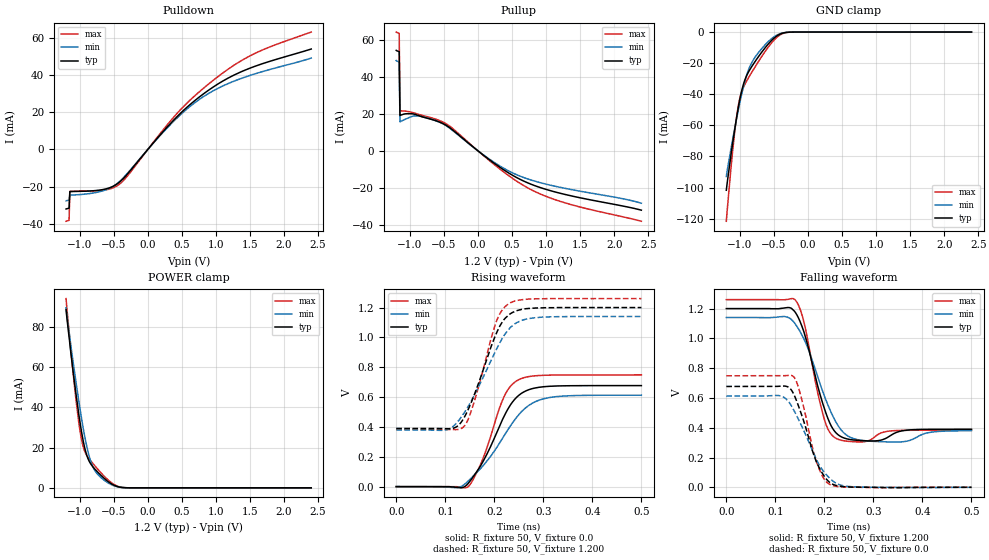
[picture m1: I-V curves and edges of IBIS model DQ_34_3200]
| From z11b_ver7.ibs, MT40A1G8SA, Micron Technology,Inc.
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| MODEL DQ_34_3200 (34 Ohm Data I/O with no ODT, 1600-3200Mbps)
[Model]   DQ_34_3200
Model_type   I/O
Vinl = 905.000mV
Vinh = 1015.000mV
Vmeas = 960.000mV
Vref = 1200.000mV
Cref = 0.0pF
Rref = 50.000Ohm
|   typ   min   max
|C_comp   0.810pF   0.760pF   0.860pF
C_comp_pullup   0.4050pF   0.3800pF   0.4300pF
C_comp_pulldown   0.4050pF   0.3800pF   0.4300pF
[Model Spec]
| Timing spec test load voltage corners
Vref   1.2000V   1.1400V   1.2600V
| Dynamic Overshoot Parameters from DDR4 Specification
|D_overshoot_ampl_h   0.40   NA   NA
|D_overshoot_ampl_l   0.40   NA   NA
|D_overshoot_area_h   0.0800n   NA   NA
|D_overshoot_area_l   0.0800n   NA   NA
[Voltage Range]   1.2000V   1.1400V   1.2600V
| Junction Temperature (Ambient temp is 35C typ, 95C min, 0C max)
[Temperature Range]   50.0   110.0   0.0
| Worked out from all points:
|   slope of the pulldown table from 0 to 0.18 V, typ, clamps not added: 23.2 ohm
|   slope of the pullup table from 0 to 0.18 V, typ, clamps not added: 35.1 ohm
|   GND clamp passes 1 mA (typ) near -0.39 V on its own axis
|   POWER clamp passes 1 mA (typ) near -0.48 V on its own axis
|   rising waveform, R_fixture 50, V_fixture 0.0: 20-80 % time 60.5ps typ, 79.7ps min, 47.2ps max; typ from 0 V to 0.677 V
|   falling waveform, R_fixture 50, V_fixture 1.200: 20-80 % time 39ps typ, 50.4ps min, 31.7ps max; typ from 1.2 V to 0.39 V
|   rising waveform, R_fixture 50, V_fixture 1.200: 20-80 % time 54.3ps typ, 69.6ps min, 43.8ps max; typ from 0.39 V to 1.2 V
|   falling waveform, R_fixture 50, V_fixture 0.0: 20-80 % time 41.1ps typ, 52.9ps min, 33.2ps max; typ from 0.677 V to 0 V
[Pulldown]
|   Voltage   I(typ)   I(min)   I(max)
-1.2V     -32.14mA   -27.78mA   -38.76mA
-1.156V   -31.69mA   -27.3mA    -38.27mA
-1.145V   -22.74mA   -24.67mA   -22.62mA
-698.2mV  -21.88mA   -22.71mA   -22.17mA
-545.5mV  -20.46mA   -20.64mA   -21.17mA
-414.5mV  -17.59mA   -17.27mA   -18.66mA
-294.5mV  -13.07mA   -12.67mA   -14.11mA
458.2mV   18.75mA    17.99mA    20.61mA
752.7mV   28.18mA    26.87mA    30.99mA
1.047V    35.72mA    33.3mA     39.78mA
1.571V    44.84mA    40.76mA    51.79mA
2.4V      54.19mA    49.29mA    63.35mA
[GND_clamp]
|   Voltage   I(typ)   I(min)   I(max)
-1.2V     -101.7mA   -92.84mA   -121.7mA
-1.135V   -79.96mA   -75.84mA   -88.92mA
-1.08V    -63.49mA   -62.76mA   -65.41mA
-1.036V   -51.56mA   -52.83mA   -50.65mA
-992.7mV  -41.38mA   -43.57mA   -41.02mA
-927.3mV  -30.76mA   -31.6mA    -33.57mA
-872.7mV  -25.55mA   -24.13mA   -29.29mA
-818.2mV  -21.61mA   -19.01mA   -25.29mA
-621.8mV  -9.66mA    -7.8mA     -11.96mA
-436.4mV  -1.915mA   -1.476mA   -2.607mA
-229.1mV  -17.62uA   -20.1uA    -21.35uA
2.4V      0A         0A         0A
[Pullup]
|   Voltage   I(typ)   I(min)   I(max)
-1.2V     54.34mA    48.83mA    64.24mA
-1.156V   53.69mA    48.13mA    63.57mA
-1.145V   19.17mA    15.69mA    21.61mA
-916.4mV  19.61mA    18.89mA    20.24mA
-567.3mV  15.61mA    15.52mA    16.42mA
-370.9mV  11.29mA    10.99mA    12.08mA
0V        840nA      835.9nA    929.5nA
327.3mV   -9.01mA    -8.316mA   -9.985mA
589.1mV   -14.86mA   -13.25mA   -16.89mA
861.8mV   -19.2mA    -16.69mA   -22.46mA
1.418V    -24.76mA   -21.28mA   -29.6mA
2.4V      -32.09mA   -28.34mA   -38.11mA
[POWER_clamp]
|   Voltage   I(typ)   I(min)   I(max)
-1.2V     88.79mA    89.61mA    94.2mA
-1.135V   68.71mA    72.12mA    70.03mA
-1.058V   47.63mA    53.55mA    44.95mA
-1.004V   34.46mA    41.11mA    30.27mA
-960mV    25.41mA    31.92mA    21.99mA
-894.5mV  16.02mA    20.41mA    16.03mA
-850.9mV  12.63mA    14.54mA    13.97mA
-807.3mV  10.5mA     10.53mA    12.15mA
-709.1mV  6.91mA     5.769mA    8.279mA
-545.5mV  2.224mA    1.735mA    2.842mA
-305.5mV  24.75uA    26.66uA    31.49uA
2.4V      0A         0A         0A
[Ramp]
|   typ   min   max
dV/dt_r   406.22m/60.49p   367.64m/79.70p   449.27m/47.23p
dV/dt_f   486.12m/38.95p   456.09m/50.39p   526.01m/31.70p
R_load = 50
[Rising Waveform]
R_fixture = 50
V_fixture = 0.0
|   Time   V(typ)   V(min)   V(max)
0s        2.16uV     7.745uV    1.281uV
124ps     -5.863mV   -6.685mV   -787.9uV
147ps     22.02mV    37.71mV    729.1uV
176ps     161.9mV    135.5mV    180.1mV
221ps     478.1mV    346.1mV    610mV
235ps     557.2mV    416.9mV    679.8mV
252ps     617mV      489.5mV    719.8mV
280ps     658.7mV    563.2mV    741.7mV
317ps     673.1mV    599.2mV    747.5mV
500ps     677mV      612.7mV    748.8mV
[Falling Waveform]
R_fixture   = 50
V_fixture   = 1.200
V_fixture_min = 1.140
V_fixture_max = 1.260
|   Time   V(typ)   V(min)   V(max)
0s        1.2V       1.14V      1.26V
118ps     1.204V     1.147V     1.259V
142ps     1.168V     1.09V      1.253V
158ps     1.046V     997.9mV    1.113V
200ps     528.4mV    612.9mV    455mV
225ps     361.3mV    429.4mV    326.6mV
252ps     321mV      337.1mV    307.8mV
297ps     311mV      308.7mV    324.4mV
366ps     382.9mV    308.6mV    382.8mV
500ps     389.8mV    379.8mV    383.3mV
[Rising Waveform]
R_fixture   = 50
V_fixture   = 1.200
V_fixture_min = 1.140
V_fixture_max = 1.260
|   Time   V(typ)   V(min)   V(max)
0s        389.8mV    380mV      383.3mV
104ps     387.7mV    381.8mV    383.2mV
124ps     403mV      429.7mV    382.2mV
139ps     465.1mV    496.3mV    405.9mV
160ps     622.1mV    616.5mV    578.5mV
205ps     1.032V     924.6mV    1.113V
217ps     1.106V     996.7mV    1.187V
234ps     1.161V     1.07V      1.234V
290ps     1.198V     1.134V     1.259V
500ps     1.2V       1.14V      1.26V
[Falling Waveform]
R_fixture = 50
V_fixture = 0.0
|   Time   V(typ)   V(min)   V(max)
0s        677.1mV    612.8mV    748.8mV
109ps     679mV      614.8mV    748.3mV
126ps     673.4mV    579.2mV    751.6mV
137ps     628.9mV    522.1mV    743.5mV
151ps     511.1mV    429.7mV    624.8mV
184ps     169.1mV    184mV      170.4mV
198ps     82.68mV    108.4mV    63.01mV
212ps     30.06mV    56.98mV    17.77mV
258ps     1.401mV    3.503mV    831.8uV
500ps     7.466uV    -37.9uV    6.335uV
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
